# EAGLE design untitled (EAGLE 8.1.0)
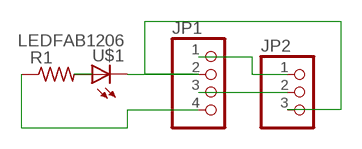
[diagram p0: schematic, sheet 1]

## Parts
JP1  PINHD-1X4  [1X04]
JP2  PINHD-1X3  [1X03]
R1  RES-US1206FAB  [R1206FAB]
U$1  LEDFAB1206  [LED1206FAB]

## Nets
N$1: R1.2 U$1.1(A)
N$2: JP1.4 R1.1
N$3: JP1.2 JP2.3 U$1.2(C)
N$4: JP1.3 JP2.2
N$5: JP1.1 JP2.1

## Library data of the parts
JP1 = pinhead:PINHD-1X4: PIN HEADER
JP2 = pinhead:PINHD-1X3: PIN HEADER
R1 = fab:RES-US: Resistor (US Symbol)
U$1 = fab:LED: LED

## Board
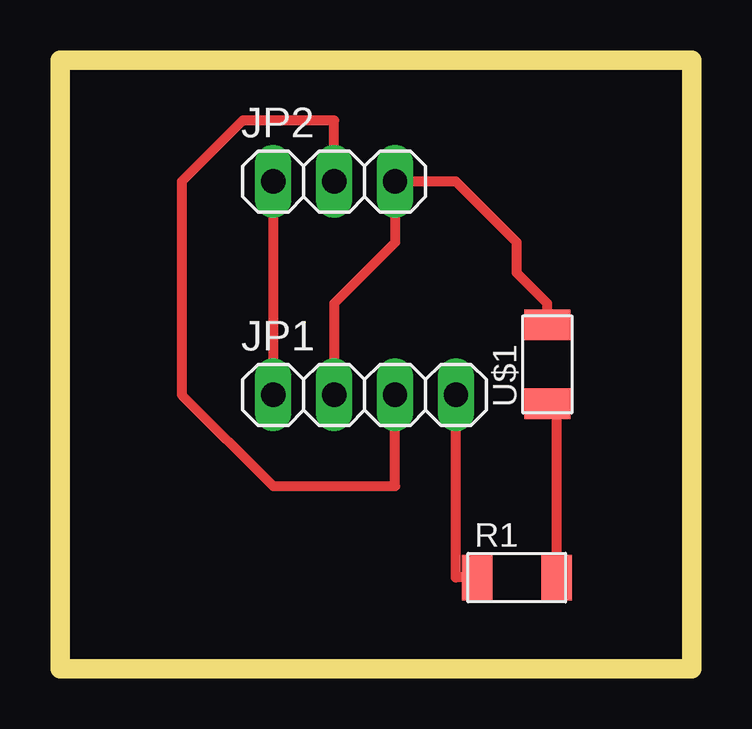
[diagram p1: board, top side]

Size 26.34 x 25.39 mm. Coordinates in mm from the lower left corner, seen from the top.
Outline: 0,0 26.34,0 26.34,25.39 0,25.39 0,0
Copper layers (1*16): Top 0.035mm / dielectric 1.5mm / Bottom 0.035mm
Design rules "default *": minimum track width 16mil, minimum drill 24mil, track to track 16mil, track to pad 16mil, pad to pad 16mil, via to via 16mil, smd to smd 8mil, copper to edge 40mil, drill to drill 8mil, minimum pad ring 10mil, minimum via ring 8mil, stop-mask expansion 4mil, vias tented up to drill 0mil, thermal gap 10mil

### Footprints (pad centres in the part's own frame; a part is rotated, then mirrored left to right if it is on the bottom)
1X04 = drill 1.016 long: 1 -3.81,0; 2 -1.27,0; 3 1.27,0; 4 3.81,0
1X03 = drill 1.016 long: 1 -2.54,0; 2 0,0; 3 2.54,0
R1206FAB = smd 1.27 x 1.905: 1 -1.651,0; 2 1.651,0
LED1206FAB = smd 1.27 x 1.905: 1 -1.651,0; 2 1.651,0

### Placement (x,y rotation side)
JP1  12.7,11.43 0 top
JP2  11.43,20.32 0 top
R1  19.05,3.81 0 top
U$1  20.32,12.7 90 top

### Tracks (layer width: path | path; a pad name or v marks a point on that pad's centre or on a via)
N$1
  Top 0.406: U$1.1 20.7,11.05 R1.2
N$2
  Top 0.406: R1.1 16.51,3.81 JP1.4
N$3
  Top 0.406: JP1.2 11.43,15.24 13.97,17.78 JP2.3 16.51,20.32 19.05,17.78 19.05,16.51 20.32,15.24 U$1.2
N$4
  Top 0.406: JP2.2 11.43,22.86 7.62,22.86 5.08,20.32 5.08,11.43 8.89,7.62 13.97,7.62 JP1.3
N$5
  Top 0.406: JP2.1 JP1.1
